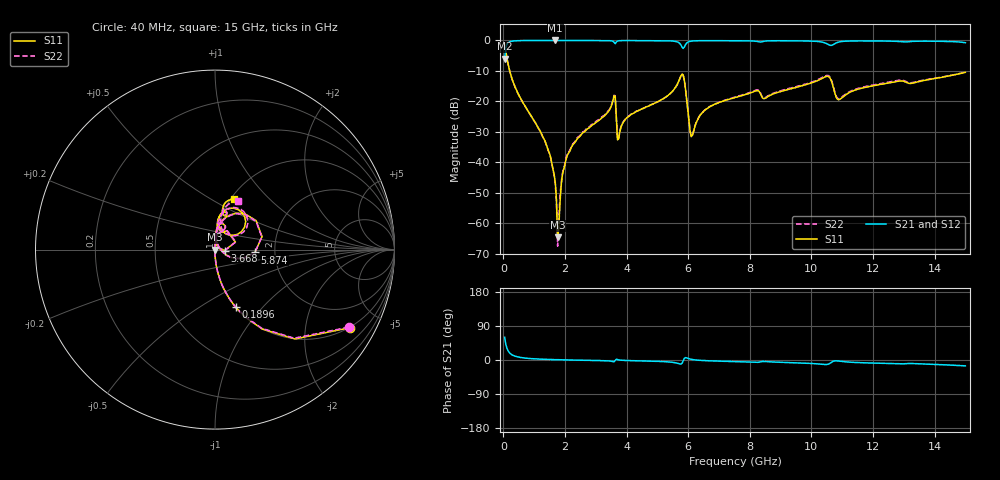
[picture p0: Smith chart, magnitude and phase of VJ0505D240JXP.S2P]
! VJ0505D240JXP
! MLCC placed on 25 mil thick microstrip substrate in series configuraton.
! DATE 06/29/2018  09:11
! CORRECTED  DATA
# GHz  S  MA  R  50.00
!  FREQ  S11M  S11A  S21M  S21A  S12M  S12A  S22M  S22A
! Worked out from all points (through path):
!   401 points, 40 MHz to 15 GHz, reference 50 ohm
!   highest |S21| = -0.01 dB at 1.686 GHz (marker M1); lowest = -6.0 dB at 40 MHz (marker M2)
!   group delay of S21, straight-line fit = 3.43 ps
!   lowest |S11| = -64.7 dB at 1.76 GHz (marker M3), VSWR 1.00, Z = 50 - j0.0549 ohm
!   |S11| at or under -10 dB: 206.5 MHz to end of sweep
!   |S22| runs from -67.6 to -1.3 dB; largest |S21 - S12| = 0.0027
!   S11 on the Smith chart (normalised r, x): 40 MHz: 0.98, -3.47; 189.6 MHz: 1.00, -0.72; 3.668 GHz: 1.11, -0.01; 5.874 GHz: 1.57, -0.05; 15 GHz: 1.03, +0.64
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0.04  0.8686 -30.0  0.5013 59.9  0.5011 60.0  0.8612 -30.1
0.1896  0.3411 -70.4  0.9394 20.0  0.9402 19.9  0.3381 -70.4
1.4238  0.0175 -90.6  0.9981 1.6  0.9988 1.6  0.01728 -91.0
1.6108  0.00766 -92.0  0.9981 1.1  0.9987 1.2  0.007407 -93.6
1.6856  0.004614 -92.6  0.9986 0.9  0.9985 1.0  0.004402 -95.1
1.7604  0.0005823 -109.4  0.9983 0.7  0.9982 0.8  0.0004178 -140.1
1.8352  0.002032 97.6  0.9968 0.6  0.9982 0.6  0.002614 95.7
2.0222  0.01043 90.7  0.9979 0.3  0.9981 0.3  0.01103 89.2
2.5458  0.02919 89.1  0.9964 -0.6  0.997 -0.5  0.03034 87.7
3.5556  0.1013 72.6  0.9695 -4.1  0.9699 -4.1  0.1039 72.6
3.6678  0.05446 -5.3  0.9437 2.0  0.9444 2.1  0.05538 -5.2
3.78  0.03136 76.9  0.9905 -0.1  0.9911 -0.1  0.03195 77.4
5.0516  0.101 85.4  0.9907 -3.7  0.9914 -3.6  0.1002 84.8
5.8744  0.2232 -4.0  0.7788 4.3  0.7796 4.3  0.2218 -4.6
6.1362  0.02759 44.6  0.9784 1.3  0.9789 1.3  0.02734 45.2
6.5476  0.07195 85.6  0.9912 -1.7  0.9919 -1.6  0.07268 84.4
7.52  0.1155 85.3  0.9893 -4.2  0.9901 -4.1  0.1179 84.8
10.0258  0.2024 80.7  0.9724 -9.3  0.974 -9.2  0.2084 78.3
10.5494  0.2558 54.0  0.8576 -10.9  0.8581 -10.9  0.2648 51.8
10.9234  0.1079 64.1  0.9498 -3.2  0.9503 -3.2  0.1107 60.9
12.5316  0.2009 79.9  0.9738 -9.4  0.9747 -9.4  0.2073 78.8
15  0.2986 69.7  0.9162 -15.5  0.9163 -15.5  0.3008 64.5
